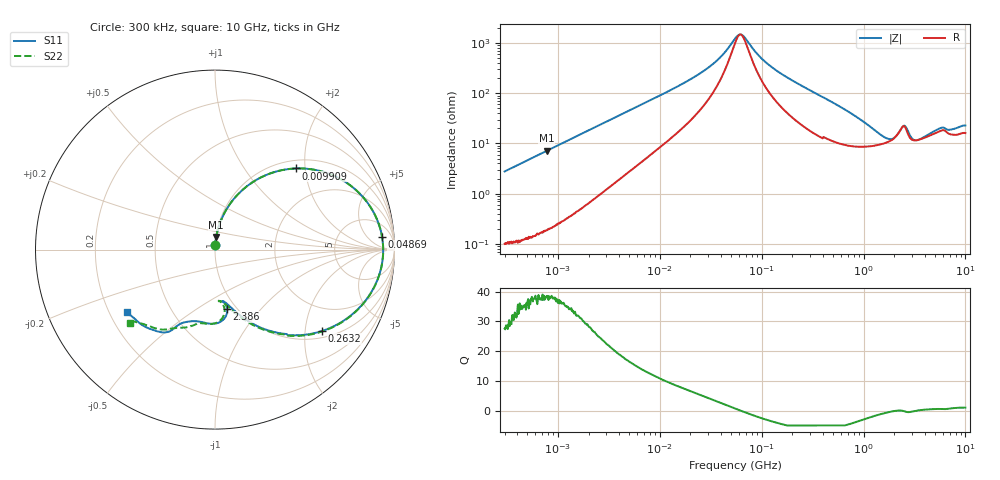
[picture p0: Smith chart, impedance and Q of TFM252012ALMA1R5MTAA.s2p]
! S-Parameter Data Generated by TDK Corporation
! Copyright(C) 2019 TDK Corporation.
! All Rights Reserved.
! TDK P/N: TFM252012ALMA1R5MTAA (Inductor)
! Property: L=1.5uH at 1MHz
! Size(LxWxT): 2.5x2x1.2mm
! Model Type: s2p (Touchstone File Format Version 1.0)
! Frequency: DC=Yes Start=0.3MHz Stop=10000MHz 802points Log-sweep
! Model Generated on May 10, 2019
! Port Assignments:
!  1 ---@@@--- 2
! Applicable Conditions:
!  Temperature = 25 degC
!  DC Bias Current = 0 A
!  Small Signal Operation
! Terms and conditions regarding TDK Simulation Models
! (1)This simulation model is being provided solely for informational purposes. Please refer to the specifications of the products in terms of detailed characteristics of such products.
! (2)In no event shall TDK Corporation of any of its subsidiaries be liable for any loss or damage arising, directly or indirectly,
!  From any information contained in this simulation model, including, but not limited to loss or damages arising from any inaccuracies, omissions or errors in connection with such information.
! (3)Any and all copyrights on this simulation model are owned by TDK Corporation.
!  Duplication or redistribution of this simulation model without prior written permission from TDK Corporation is prohibited.
! (4)This simulation model is subject to any modification or change without any prior notice.
! (5)Neither TDK Corporation nor any of its subsidiaries shall make any warranty, express or implied,
!  Including but not limited to the correctness, implied warranties of merchantability and fitness for a particular purpose with respect to this simulation models.
! (6)The use of this simulation model shall be deemed to have consented to the terms and conditions hereof.
# Hz S MA R 50
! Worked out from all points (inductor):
!   801 points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, 300 kHz to 10 GHz, reference 50 ohm
!   read as one part in series: L = 1.47 uH near 318.3 kHz
!   highest Q = 38.4 at 777.3 kHz (marker M1), where L = 1.46 uH
!   self-resonance near 61.93 MHz
!   S11 on the Smith chart (normalised r, x): 300 kHz: 1.00, +0.06; 9.909 MHz: 1.17, +1.78; 48.69 MHz: 14, +15; 263.2 MHz: 1.19, -2.47; 2.386 GHz: 0.91, -0.67; 10 GHz: 0.27, -0.30
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300000  0.02763 86.6  0.9985 -1.6  0.9983 -1.6  0.02792 87.0
777328  0.07108 84.4  0.9956 -4.1  0.9957 -4.1  0.07124 84.5
1713600  0.1541 79.3  0.983 -8.9  0.983 -8.9  0.1541 79.3
4301371  0.3557 66.0  0.9151 -20.9  0.9152 -20.9  0.3557 66.0
9671944  0.6285 45.9  0.7229 -38.9  0.723 -38.9  0.6285 45.9
9909464  0.6368 45.2  0.7147 -39.5  0.7148 -39.5  0.6367 45.2
2.599165e7  0.8802 18.6  0.3329 -60.1  0.333 -60.1  0.8802 18.6
3.686242e7  0.9187 10.4  0.1998 -61.2  0.1998 -61.2  0.9188 10.4
4.868606e7  0.9337 4.2  0.1066 -50.0  0.1066 -50.0  0.934 4.2
5.477226e7  0.9363 1.7  0.07642 -33.4  0.07644 -33.4  0.9366 1.6
6.481723e7  0.9365 -1.9  0.06525 12.5  0.06526 12.5  0.9369 -2.0
1.177683e8  0.9021 -15.3  0.244 58.1  0.2439 58.1  0.903 -15.4
2.631947e8  0.75 -37.2  0.5535 43.7  0.5535 43.7  0.7513 -37.4
3.126428e8  0.7006 -42.4  0.6169 39.0  0.6169 39.0  0.702 -42.7
7.497801e8  0.4219 -66.6  0.8333 12.9  0.8334 12.9  0.4231 -67.4
1.767019e9  0.2903 -81.7  0.8595 -12.8  0.8595 -12.8  0.2881 -84.5
2.38587e9  0.3368 -78.4  0.7765 -22.5  0.7766 -22.5  0.3263 -81.0
2.720446e9  0.4129 -90.8  0.7767 -21.0  0.7768 -21.0  0.4129 -91.4
3.598403e9  0.4178 -107.4  0.7891 -32.5  0.7891 -32.5  0.4291 -104.4
5.445625e9  0.4766 -116.6  0.701 -49.6  0.701 -49.7  0.4857 -116.0
6.576072e9  0.5494 -123.1  0.6489 -56.8  0.6489 -56.8  0.5493 -126.9
1e10  0.601 -144.8  0.5493 -80.3  0.5495 -80.4  0.6273 -139.4
